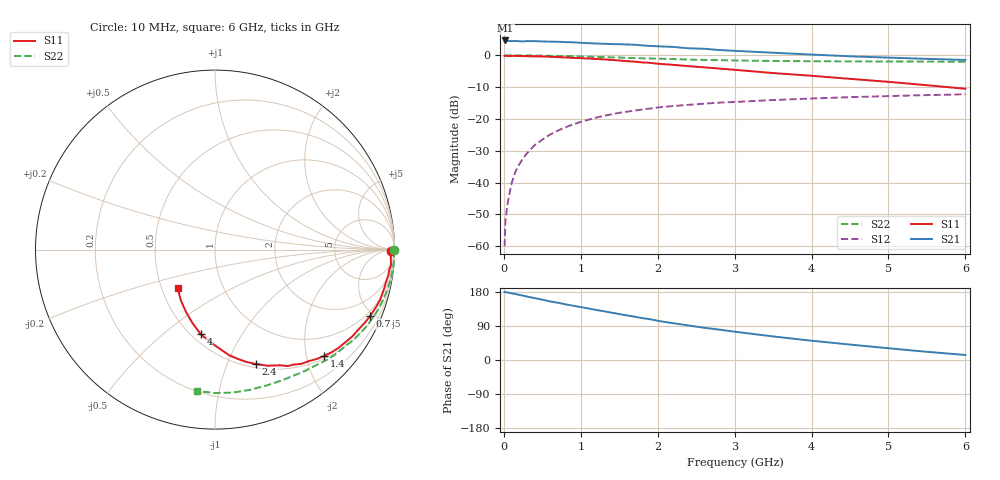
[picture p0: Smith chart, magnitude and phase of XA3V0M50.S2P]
! SIEMENS Discrete & RF Semiconductors
! BFY180
! Si NPN RF Bipolar Junction Transistor in MICRO-X
! VCE = 3 V  IC = 0.5 mA
! Common Emitter S-Parameters:  May  1997
# GHz  S  MA  R  50
!  f  S11  S21  S12  S22
! GHz  MAG  ANG  MAG  ANG  MAG  ANG  MAG  ANG
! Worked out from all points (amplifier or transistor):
!   36 points, 10 MHz to 6 GHz, reference 50 ohm
!   highest |S21| = 4.7 dB at 20 MHz (marker M1)
!   |S21| within 3 dB of that: start of sweep to 2.796 GHz
!   unconditionally stable (mu >= 1): 5.527 GHz to end of sweep
!   at 250 MHz: K = 0.05, MSG = 18.4 dB, |S12| = -32.4 dB
!   at 1.4 GHz: K = 0.40, MSG = 11.0 dB, |S12| = -18.5 dB
!   at 6 GHz: K = 1.02, MAG = 4.6 dB, |S12| = -12.2 dB
!   S11 on the Smith chart (normalised r, x): 10 MHz: 92, -24; 700 MHz: 0.75, -4.76; 1.4 GHz: 0.55, -2.35; 2.4 GHz: 0.54, -1.27; 4 GHz: 0.56, -0.68; 6 GHz: 0.61, -0.29
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0.01  0.9798 -0.3  1.665 179.8  0.001 98.8  1 -0.2
0.02  0.9844 -0.6  1.718 179.0  0.0025 91.8  0.9999 -0.4
0.05  0.9785 -1.5  1.685 178.0  0.0048 88.1  0.9988 -1.1
0.1  0.9814 -3.2  1.678 176.1  0.0097 86.8  0.9973 -2.3
0.15  0.9842 -5.1  1.688 174.1  0.0148 86.7  0.9999 -3.4
0.2  0.9769 -6.7  1.671 171.8  0.0193 86.1  0.9972 -4.6
0.3  0.9713 -10.0  1.679 167.4  0.0289 82.5  0.9951 -6.8
0.4  0.9666 -13.1  1.677 163.4  0.0387 80.2  0.9936 -9.0
0.7  0.9399 -23.2  1.64 151.2  0.0655 72.0  0.9799 -15.7
0.9  0.9146 -29.2  1.608 143.3  0.0821 66.9  0.9683 -20.1
1.1  0.8915 -35.3  1.557 135.9  0.0974 62.3  0.9543 -24.2
1.4  0.8489 -44.3  1.506 125.0  0.1184 55.5  0.9315 -30.3
1.7  0.7972 -53.0  1.472 114.2  0.1355 49.7  0.9055 -35.9
2.2  0.7108 -65.6  1.36 97.1  0.1599 40.7  0.8758 -44.4
2.4  0.6775 -70.2  1.293 91.2  0.1671 37.8  0.8604 -47.6
2.6  0.6492 -74.5  1.273 85.2  0.1737 35.1  0.8499 -50.4
3  0.5937 -82.4  1.18 74.7  0.1853 29.7  0.8327 -56.2
3.5  0.5278 -91.0  1.102 62.2  0.1988 24.2  0.8184 -62.8
4  0.4779 -99.6  1.031 50.9  0.21 18.9  0.8094 -69.4
4.5  0.4278 -107.1  0.968 40.7  0.2203 14.3  0.8052 -76.2
5.5  0.3398 -124.2  0.882 21.6  0.2375 5.2  0.7991 -90.1
6  0.2988 -134.0  0.849 13.2  0.2445 0.3  0.7939 -97.1
